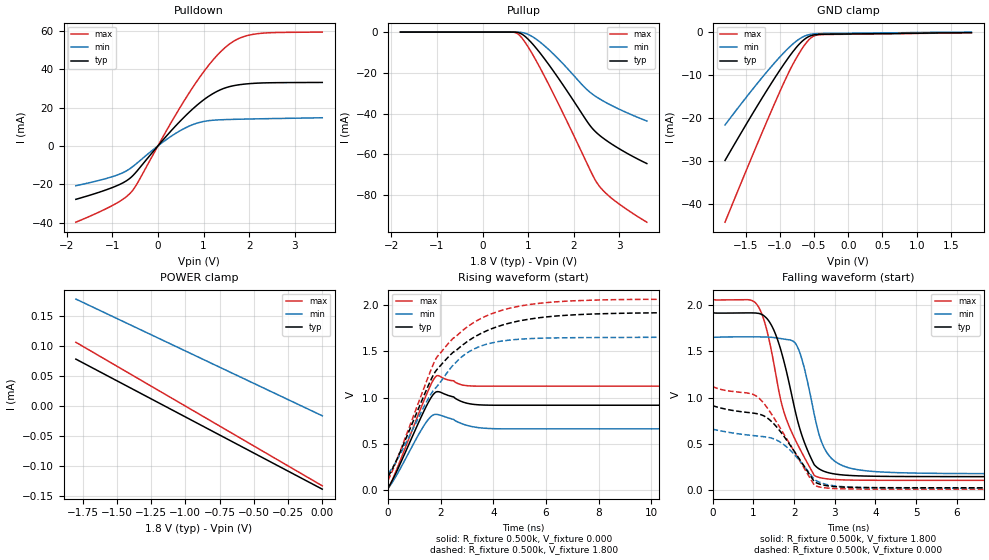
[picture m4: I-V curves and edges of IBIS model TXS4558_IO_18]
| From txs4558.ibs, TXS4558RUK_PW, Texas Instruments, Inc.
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[Model]   TXS4558_IO_18
Model_type  I/O
Vinl=0.54
Vinh=1.26
Enable   Active-Low
Vref =   0
Rref =   500
Cref =   1p
Vmeas =   0.9
| variable   typ   min   max
C_comp   4.08pF   1.40pF   6.16pF
| C_pullup   2.14pF   0.06pF   3.54pF
| C_pulldown   3.21pF   1.48pF   5.21pF
| C_tri-state   4.08pF   1.40pF   6.16pF
[Temperature Range]   40   100   -40
| Ambient temperature   25   85   -40
[Voltage range]   1.8   1.65   1.95
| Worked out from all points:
|   slope of the pulldown table from 0 to 0.27 V, typ, clamps not added: 36.8 ohm
|   GND clamp passes 1 mA (typ) near -0.57 V on its own axis
|   rising waveform, R_fixture 0.500k, V_fixture 0.000: 20-80 % time 844ps typ, 732ps min, 926ps max; typ from 0.024 V to 0.918 V
|   falling waveform, R_fixture 0.500k, V_fixture 1.800: 20-80 % time 628ps typ, 496ps min, 721ps max; typ from 1.92 V to 0.144 V
|   rising waveform, R_fixture 0.500k, V_fixture 1.800: 20-80 % time 2.23ns typ, 1.88ns min, 2.06ns max; typ from 0.144 V to 1.92 V
|   falling waveform, R_fixture 0.500k, V_fixture 0.000: 20-80 % time 878ps typ, 840ps min, 933ps max; typ from 0.918 V to 0.024 V
[GND Clamp]
| TXS4558_IO_18
|   Voltage   I(typ)   I(min)   I(max)
-1.8V     -29.85mA   -21.6mA    -44.21mA
-1.285V   -16.03mA   -11.09mA   -24.38mA
-1.075V   -10.71mA   -7.135mA   -16.59mA
-915mV    -6.893mA   -4.38mA    -10.92mA
-815mV    -4.701mA   -2.861mA   -7.683mA
-705mV    -2.628mA   -1.511mA   -4.626mA
-615mV    -1.403mA   -795.6uA   -2.531mA
-540mV    -808.4uA   -496.2uA   -1.292mA
-470mV    -583.5uA   -374.8uA   -739.1uA
-375mV    -509uA     -323.1uA   -575uA
1.8V      -138.4uA   106.5pA    -152.8uA
[POWER Clamp]
| TXS4558_IO_18
|   Voltage   I(typ)   I(min)   I(max)
-1.8V     78.25uA    178.3uA    106.3uA
-1.17V    2.408uA    110.2uA    22.59uA
-1.16V    1.204uA    109.1uA    21.26uA
-16.28fV  -138.4uA   -16.21uA   -132.9uA
[Pulldown]
| TXS4558_IO_18
|   Voltage   I(typ)   I(min)   I(max)
-1.8V     -27.79mA   -20.7mA    -39.69mA
-945mV    -21.12mA   -15.56mA   -30.31mA
-725mV    -18.61mA   -13.39mA   -26.99mA
-575mV    -15.99mA   -11.13mA   -23.7mA
-440mV    -12.49mA   -8.547mA   -18.91mA
130mV     3.68mA     2.408mA    5.641mA
605mV     15.78mA    9.475mA    24.72mA
1.12V     26.02mA    13.21mA    42.32mA
1.545V    30.76mA    13.79mA    52.69mA
1.82V     32.02mA    13.96mA    56.47mA
2.155V    32.69mA    14.13mA    58.4mA
3.6V      33.1mA     14.7mA     59.32mA
[Pullup]
| TXS4558_IO_18
|   Voltage   I(typ)   I(min)   I(max)
-1.8V     0A         0A         0A
655mV     -2.319uA   -93.15nA   -26.22uA
780mV     -247.9uA   -22.48uA   -1.008mA
870mV     -1.122mA   -230.5uA   -3.103mA
985mV     -3.205mA   -1.011mA   -6.809mA
1.3V      -11.42mA   -5.634mA   -19.24mA
1.66V     -22.57mA   -13.14mA   -35.09mA
2.32V     -44.78mA   -28.86mA   -65.89mA
2.52V     -49.8mA    -32.14mA   -74.36mA
2.665V    -52.38mA   -34.06mA   -78.22mA
2.87V     -55.49mA   -36.47mA   -82.25mA
3.6V      -64.48mA   -43.61mA   -93.23mA
[Ramp]
| TXS4558_IO_18
| variable   typ   min   max
dV/dt_r   0.62/9.88E-10   0.48/9.19E-10   0.74/1.03E-09
dV/dt_f   1.04/6.29E-10   0.89/5.01E-10   1.15/7.23E-10
R_load = 500
[Rising Waveform]
R_fixture = 0.500k
V_fixture = 0.000
V_fixture_min = 0.000
V_fixture_max = 0.000
C_fixture = 0.000
L_fixture = 0.000
|  time   V(typ)   V(min)   V(max)
0s        23.54mV    18.87mV    8.68mV
330ps     203.2mV    163.5mV    224.5mV
1.415ns   885.5mV    719.8mV    1.004V
1.705ns   1.03V      810.5mV    1.185V
1.865ns   1.064V     817.7mV    1.238V
2.495ns   1.007V     763.1mV    1.182V
2.86ns    950.4mV    711.6mV    1.134V
3.375ns   923.4mV    677.1mV    1.124V
4.095ns   917.5mV    663mV      1.124V
24.99ns   917.5mV    662.2mV    1.124V
[Falling Waveform]
R_fixture = 0.500k
V_fixture = 1.800
V_fixture_min = 1.650
V_fixture_max = 1.950
C_fixture = 0.000
L_fixture = 0.000
|  time   V(typ)   V(min)   V(max)
0s        1.924V     1.658V     2.067V
1.13ns    1.912V     1.658V     1.979V
1.56ns    1.668V     1.647V     1.23V
1.74ns    1.41V      1.635V     859.9mV
2.01ns    889.4mV    1.6V       560.6mV
2.385ns   374.5mV    1.058V     245.4mV
2.71ns    206.5mV    482.7mV    126.5mV
3.235ns   161.1mV    255.4mV    108.8mV
4.535ns   146.1mV    187.5mV    104.5mV
24.99ns   144.3mV    175.2mV    104.2mV
[Rising Waveform]
R_fixture = 0.500k
V_fixture = 1.800
V_fixture_min = 1.650
V_fixture_max = 1.950
C_fixture = 0.000
L_fixture = 0.000
|  time   V(typ)   V(min)   V(max)
0s        144.3mV    175.2mV    104.2mV
420ps     386.6mV    367.5mV    391.7mV
1.52ns    1.126V     986mV      1.221V
1.85ns    1.302V     1.119V     1.437V
2.495ns   1.498V     1.36V      1.649V
2.965ns   1.598V     1.477V     1.757V
4.415ns   1.792V     1.616V     1.953V
6.03ns    1.874V     1.645V     2.029V
8.51ns    1.911V     1.651V     2.06V
24.99ns   1.924V     1.656V     2.067V
[Falling Waveform]
R_fixture = 0.500k
V_fixture = 0.000
V_fixture_min = 0.000
V_fixture_max = 0.000
C_fixture = 0.000
L_fixture = 0.000
|  time   V(typ)   V(min)   V(max)
0s        917.5mV    662.2mV    1.124V
935ps     835.4mV    591.8mV    1.043V
1.14ns    821.1mV    582.5mV    992.8mV
1.43ns    747.4mV    563.5mV    831.2mV
1.76ns    575.1mV    486.6mV    596.8mV
2.065ns   378.9mV    354.4mV    371.6mV
2.495ns   90.85mV    114.6mV    52.33mV
2.785ns   47.57mV    60.93mV    21.97mV
4.86ns    24.07mV    20.74mV    8.797mV
24.99ns   23.54mV    18.87mV    8.679mV
